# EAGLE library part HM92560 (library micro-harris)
MICROCONTROLLER/MEMORY DEVICE
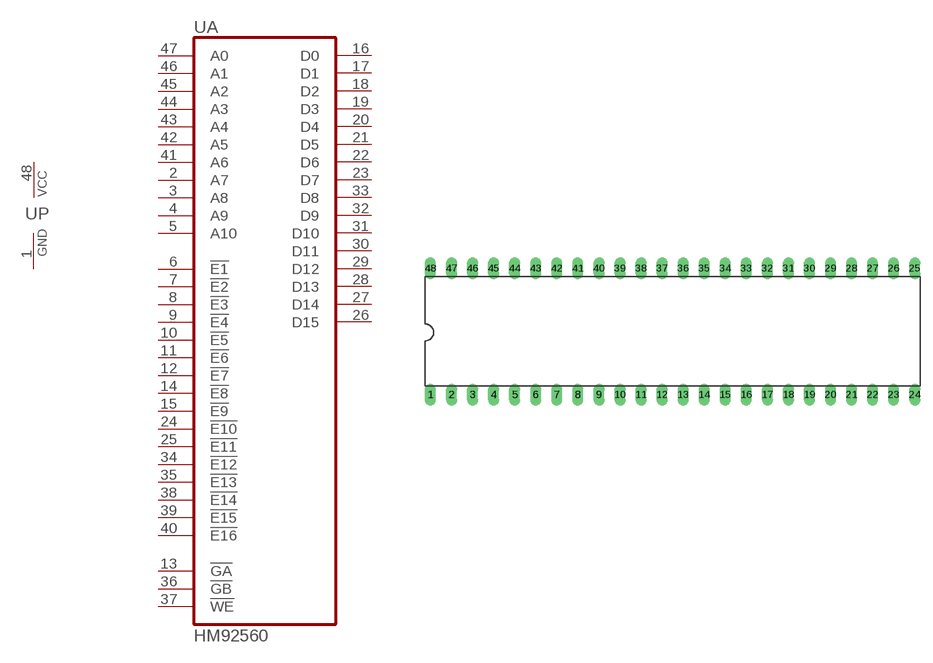
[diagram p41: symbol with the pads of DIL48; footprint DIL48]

Designator prefix U; gates A=HM92560 P=PWRN

## HM92560 (OC_FARNELL: unknown; OC_NEWARK: unknown)  [DIL48]
1  P:GND  pwr
2  A:A7  in
3  A:A8  in
4  A:A9  in
5  A:A10  in
6  A:!E1  in
7  A:!E2  in
8  A:!E3  in
9  A:!E4  in
10  A:!E5  in
11  A:!E6  in
12  A:!E7  in
13  A:!GA  in
14  A:!E8  in
15  A:!E9  in
16  A:D0
17  A:D1
18  A:D2
19  A:D3
20  A:D4
21  A:D5
22  A:D6
23  A:D7
24  A:!E10  in
25  A:!E11  in
26  A:D15
27  A:D14
28  A:D13
29  A:D12
30  A:D11
31  A:D10
32  A:D9
33  A:D8
34  A:!E12  in
35  A:!E13  in
36  A:!GB  in
37  A:!WE  in
38  A:!E14  in
39  A:!E15  in
40  A:!E16  in
41  A:A6  in
42  A:A5  in
43  A:A4  in
44  A:A3  in
45  A:A2  in
46  A:A1  in
47  A:A0  in
48  P:VCC  pwr

## Footprint DIL48 (pad centres in mm)
Dual In Line Package
drill 0.813 long: 1 -29.21,-7.62; 2 -26.67,-7.62; 3 -24.13,-7.62; 4 -21.59,-7.62; 5 -19.05,-7.62; 6 -16.51,-7.62; 7 -13.97,-7.62; 8 -11.43,-7.62; 9 -8.89,-7.62; 10 -6.35,-7.62; 11 -3.81,-7.62; 12 -1.27,-7.62; 13 1.27,-7.62; 14 3.81,-7.62; 15 6.35,-7.62; 16 8.89,-7.62; 17 11.43,-7.62; 18 13.97,-7.62; 19 16.51,-7.62; 20 19.05,-7.62; 21 21.59,-7.62; 22 24.13,-7.62; 23 26.67,-7.62; 24 29.21,-7.62; 25 29.21,7.62; 26 26.67,7.62; 27 24.13,7.62; 28 21.59,7.62; 29 19.05,7.62; 30 16.51,7.62; 31 13.97,7.62; 32 11.43,7.62; 33 8.89,7.62; 34 6.35,7.62; 35 3.81,7.62; 36 1.27,7.62; 37 -1.27,7.62; 38 -3.81,7.62; 39 -6.35,7.62; 40 -8.89,7.62; 41 -11.43,7.62; 42 -13.97,7.62; 43 -16.51,7.62; 44 -19.05,7.62; 45 -21.59,7.62; 46 -24.13,7.62; 47 -26.67,7.62; 48 -29.21,7.62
